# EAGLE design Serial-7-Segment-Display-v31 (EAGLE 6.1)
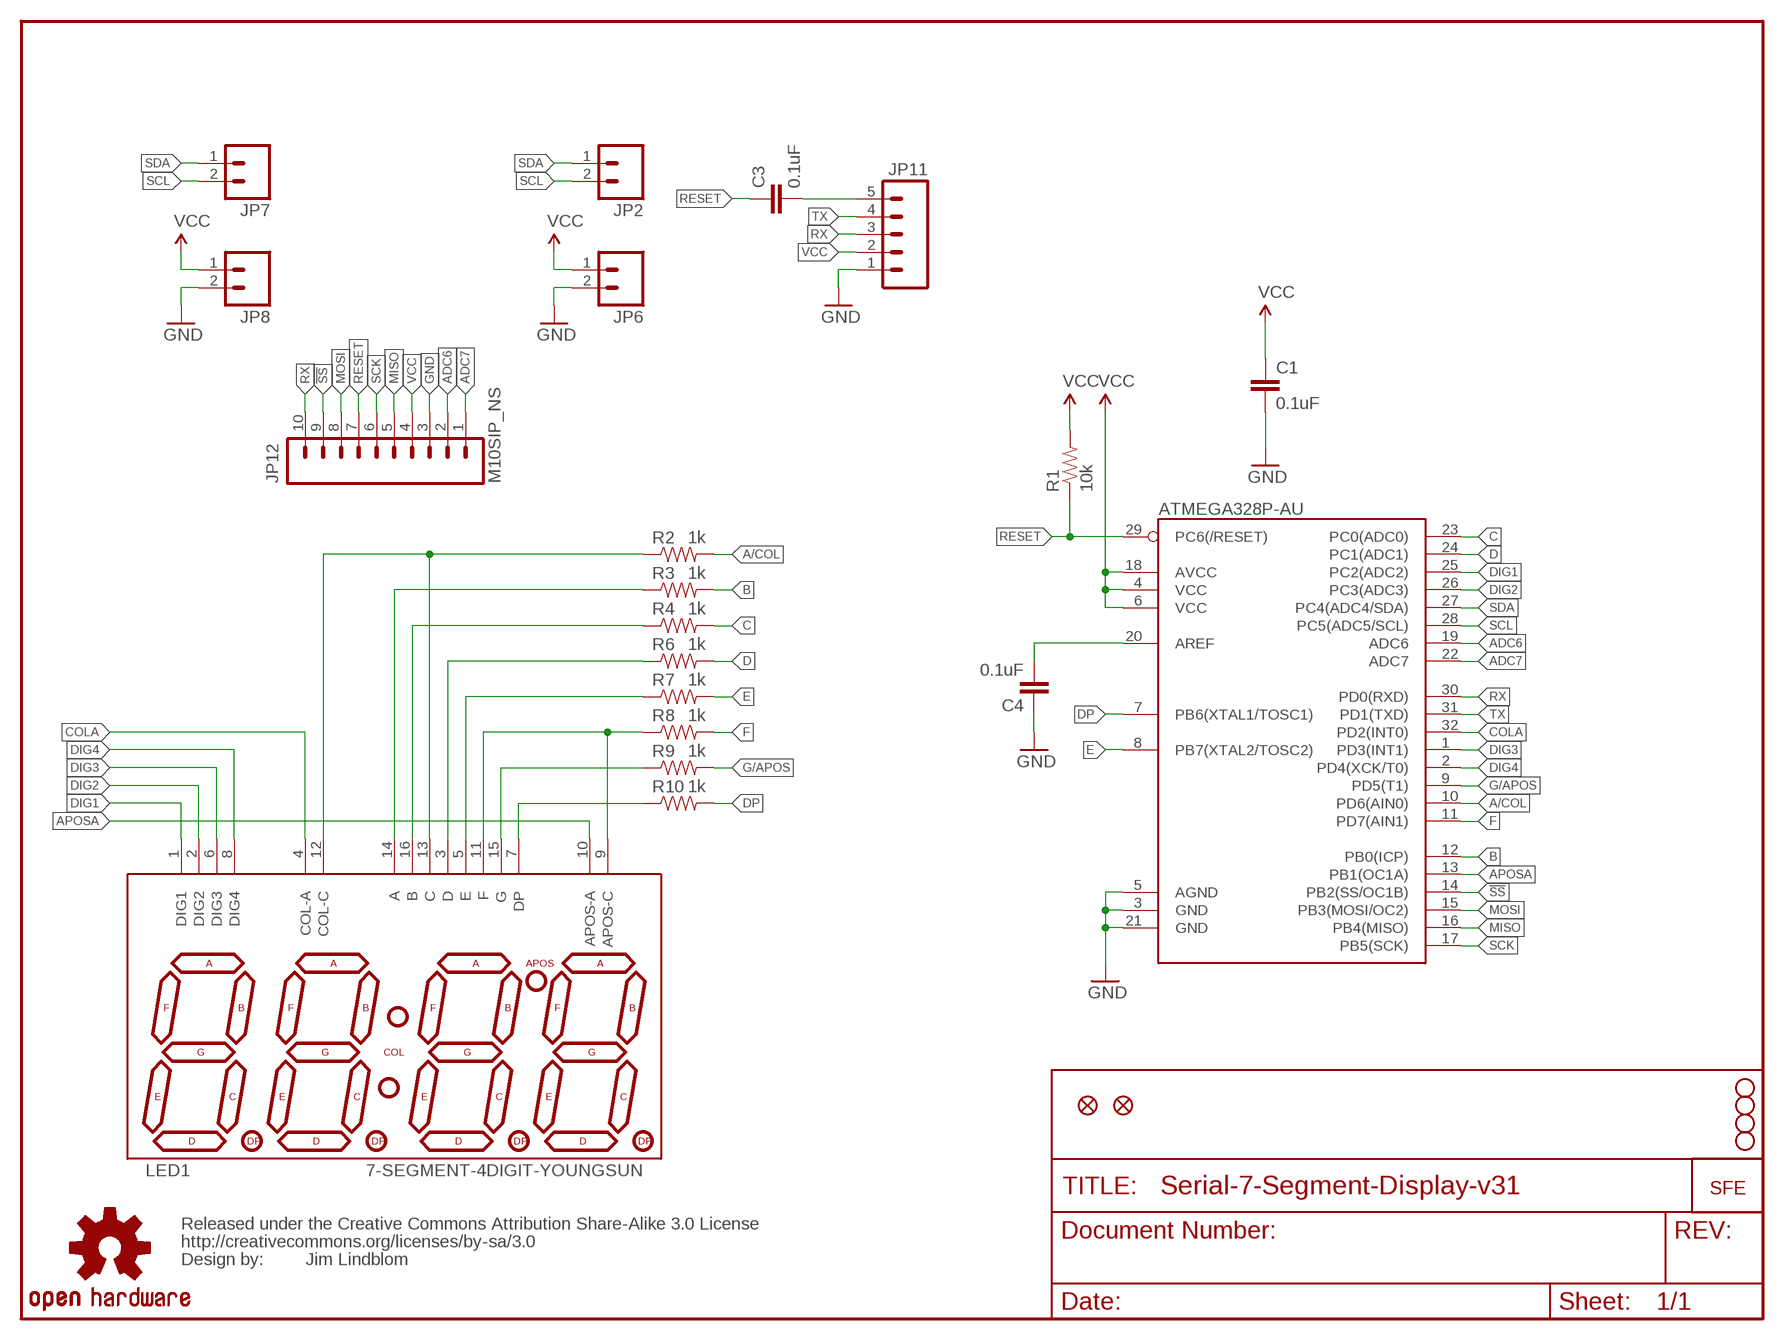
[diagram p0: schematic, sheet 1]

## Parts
ATMEGA328P-AU  ATMEGA328P-AU  ATMEGA168  [TQFP32-08]
C1  0.1uF  CAP0402-CAP  [0402-CAP]
C3  0.1uF  CAP0402-CAP  [0402-CAP]
C4  0.1uF  CAP0402-CAP  [0402-CAP]
JP1  STAND-OFF  [STAND-OFF]
JP2  M021X02_NO_SILK  [1X02_NO_SILK]
JP3  STAND-OFF  [STAND-OFF]
JP4  STAND-OFF  [STAND-OFF]
JP5  STAND-OFF  [STAND-OFF]
JP6  M021X02_NO_SILK  [1X02_NO_SILK]
JP7  M021X02_NO_SILK  [1X02_NO_SILK]
JP8  M021X02_NO_SILK  [1X02_NO_SILK]
JP9  FIDUCIALUFIDUCIAL  [MICRO-FIDUCIAL]
JP10  FIDUCIALUFIDUCIAL  [MICRO-FIDUCIAL]
JP11  M05PTH-NS  [1X05_NO_SILK]
JP12  M10SIP_NS  [1X10_NO_SILK]
LED1  7-SEGMENT-4DIGIT-YOUNGSUN  [7-SEGMENT-4DIGIT-YOUNGSUN]
R1  10k  RESISTOR0402-RES  [0402-RES]
R2  1k  RESISTOR0402-RES  [0402-RES]
R3  1k  RESISTOR0402-RES  [0402-RES]
R4  1k  RESISTOR0402-RES  [0402-RES]
R6  1k  RESISTOR0402-RES  [0402-RES]
R7  1k  RESISTOR0402-RES  [0402-RES]
R8  1k  RESISTOR0402-RES  [0402-RES]
R9  1k  RESISTOR0402-RES  [0402-RES]
R10  1k  RESISTOR0402-RES  [0402-RES]
U$1  CREATIVE_COMMONS  [CREATIVE_COMMONS]
U$2  LOGO-SFESK  [SFE-LOGO-FLAME]
U$4  OSHW-LOGOS  [OSHW-LOGO-S]

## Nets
!SS: ATMEGA328P-AU.14(PB2(SS/OC1B)) JP12.9
A/COL: ATMEGA328P-AU.10(PD6(AIN0)) R2.2
ADC6: ATMEGA328P-AU.19(ADC6) JP12.2
ADC7: ATMEGA328P-AU.22(ADC7) JP12.1
APOSA: ATMEGA328P-AU.13(PB1(OC1A)) LED1.10(APOS-A)
B: ATMEGA328P-AU.12(PB0(ICP)) R3.2
C: ATMEGA328P-AU.23(PC0(ADC0)) R4.2
COLA: ATMEGA328P-AU.32(PD2(INT0)) LED1.4(COL-A)
D: ATMEGA328P-AU.24(PC1(ADC1)) R6.2
DIG1: ATMEGA328P-AU.25(PC2(ADC2)) LED1.1(DIG1)
DIG2: ATMEGA328P-AU.26(PC3(ADC3)) LED1.2(DIG2)
DIG3: ATMEGA328P-AU.1(PD3(INT1)) LED1.6(DIG3)
DIG4: ATMEGA328P-AU.2(PD4(XCK/T0)) LED1.8(DIG4)
DP: ATMEGA328P-AU.7(PB6(XTAL1/TOSC1)) R10.2
E: ATMEGA328P-AU.8(PB7(XTAL2/TOSC2)) R7.2
F: ATMEGA328P-AU.11(PD7(AIN1)) R8.2
G/APOS: ATMEGA328P-AU.9(PD5(T1)) R9.2
GND: ATMEGA328P-AU.3(GND) ATMEGA328P-AU.5(AGND) ATMEGA328P-AU.21(GND) C1.2 C4.1 JP6.2 JP8.2 JP11.1 JP12.3
MISO: ATMEGA328P-AU.16(PB4(MISO)) JP12.5
MOSI: ATMEGA328P-AU.15(PB3(MOSI/OC2)) JP12.8
N$1: ATMEGA328P-AU.20(AREF) C4.2
N$2: LED1.7(DP) R10.1
N$3: LED1.15(G) R9.1
N$4: LED1.9(APOS-C) LED1.11(F) R8.1
N$5: LED1.5(E) R7.1
N$6: LED1.3(D) R6.1
N$8: LED1.16(B) R4.1
N$9: LED1.14(A) R3.1
N$10: LED1.12(COL-C) LED1.13(C) R2.1
N$13: C3.2 JP11.5
RESET: ATMEGA328P-AU.29(PC6(/RESET)) C3.1 JP12.7 R1.1
RX: ATMEGA328P-AU.30(PD0(RXD)) JP11.3 JP12.10
SCK: ATMEGA328P-AU.17(PB5(SCK)) JP12.6
SCL: ATMEGA328P-AU.28(PC5(ADC5/SCL)) JP2.2 JP7.2
SDA: ATMEGA328P-AU.27(PC4(ADC4/SDA)) JP2.1 JP7.1
TX: ATMEGA328P-AU.31(PD1(TXD)) JP11.4
VCC: ATMEGA328P-AU.4(VCC) ATMEGA328P-AU.6(VCC) ATMEGA328P-AU.18(AVCC) C1.1 JP6.1 JP8.1 JP11.2 JP12.4 R1.2

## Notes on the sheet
- Jim Lindblom

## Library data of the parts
ATMEGA328P-AU = SparkFun:ATMEGA168
C1 = SparkFun:CAP: Capacitor
C3 C4 = SparkFun-Passives:CAP: Capacitor
JP1 JP3-JP5 = SparkFun-Electromechanical:STAND-OFF: #4 Stand Off
JP2 JP6-JP8 = SparkFun-Connectors:M02: Header 2
JP9 JP10 = SparkFun:FIDUCIAL: Fiducial Alignment Points
JP11 = SparkFun-Connectors:M05: Header 5 Standard 5-pin 0.1" header. Use with straight break away headers (SKU : PRT-00116), right angle break away headers (PRT-00553), swiss pins (PRT-00743), machine pins (PRT-00117), and female headers (PRT-00115). Molex polarized connector foot print use with SKU : PRT-08230 with associated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
JP12 = SparkFun-Connectors:M10: Header 10 Standard 10-pin 0.1" header. Use with straight break away headers (SKU : PRT-00116), right angle break away headers (PRT-00553), swiss pins (PRT-00743), machine pins (PRT-00117), and female headers (PRT-00115).
LED1 = SparkFun:7-SEGMENT-4DIGIT-YOUNGSUN: This is a part for the 4-Digit 7-segment LEDs from Young Sun. Different from the Digikey LEDs, all 16 pins are used. The LONGPADS Variant is used for a test jig, but you may like it because there is more pad to solder to. If you are concerned about routing space, the standard works just fine though.
R1-R4 R6-R10 = SparkFun:RESISTOR: Resistor
U$1 = SparkFun:CREATIVE_COMMONS
U$2 = SparkFun:LOGO-SFE: Spark Fun Electronics PCB Logo
U$4 = SparkFun-Aesthetics:OSHW-LOGO: Open Source Hardware Logo This logo indicates the piece of hardware it is found on incorporates a OSHW license and/or adheres to the definition of open source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

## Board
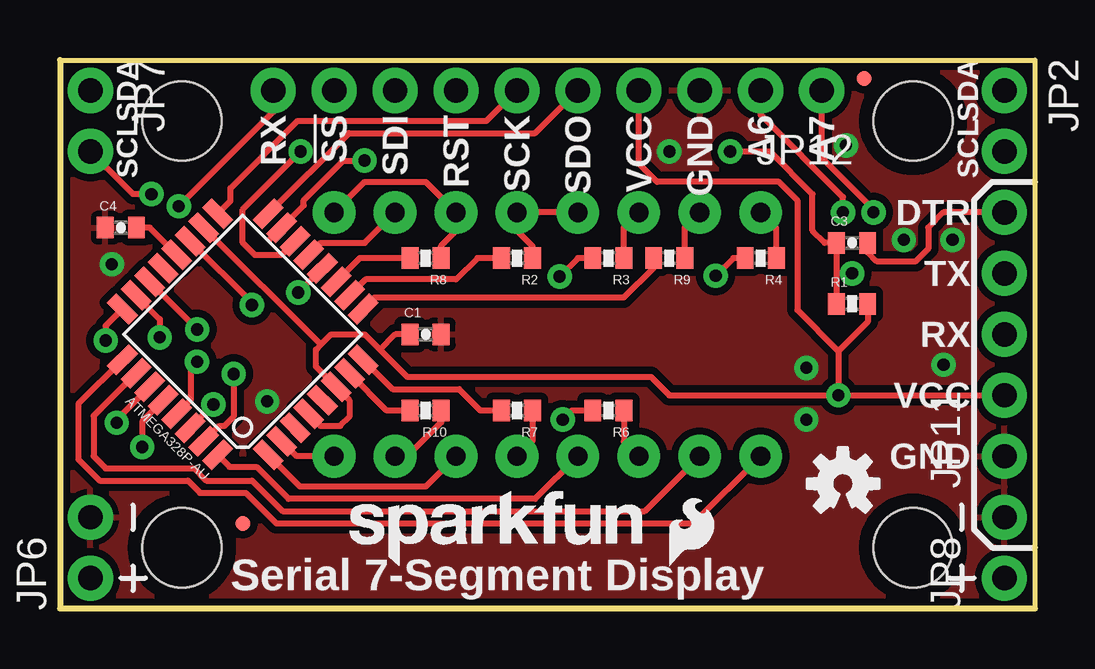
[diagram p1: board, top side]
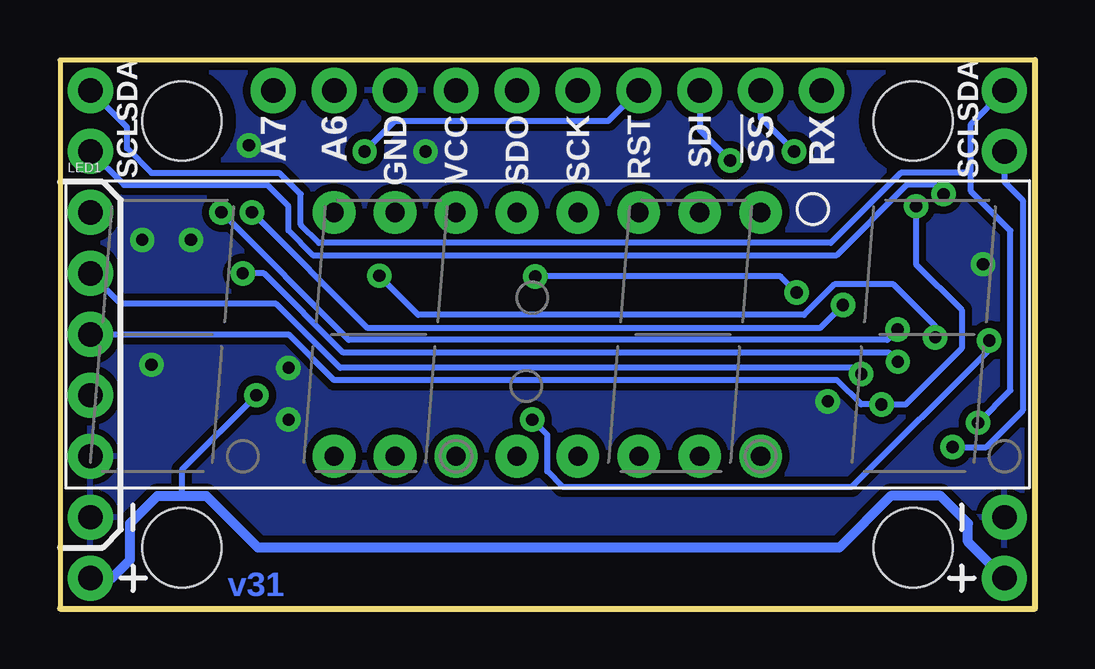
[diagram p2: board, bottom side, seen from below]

Size 40.64 x 22.86 mm. Coordinates in mm from the lower left corner, seen from the top.
Outline: 0,22.86 40.64,22.86 40.64,0 0,0 0,22.86
Copper layers (1*16): Top 0.035mm / dielectric 1.5mm / Bottom 0.035mm
Design rules: minimum track width 8mil, minimum drill 20mil, track to track 8mil, track to pad 8mil, pad to pad 8mil, via to via 8mil, smd to smd 8mil, copper to edge 8mil, drill to drill 8mil, minimum pad ring 12mil, minimum via ring 10mil, stop-mask expansion 4mil, vias tented up to drill 20mil, thermal gap 10mil

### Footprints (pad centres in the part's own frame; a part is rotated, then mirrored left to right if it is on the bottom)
TQFP32-08 = smd 1.27 x 0.559: 1 -4.293,2.8; 2 -4.293,2; 3 -4.293,1.2; 4 -4.293,0.4; 5 -4.293,-0.4; 6 -4.293,-1.2; 7 -4.293,-2; 8 -4.293,-2.8; 17 4.293,-2.8; 18 4.293,-2; 19 4.293,-1.2; 20 4.293,-0.4; 21 4.293,0.4; 22 4.293,1.2; 23 4.293,2; 24 4.293,2.8 | smd 0.559 x 1.27: 9 -2.8,-4.293; 10 -2,-4.293; 11 -1.2,-4.293; 12 -0.4,-4.293; 13 0.4,-4.293; 14 1.2,-4.293; 15 2,-4.293; 16 2.8,-4.293; 25 2.8,4.293; 26 2,4.293; 27 1.2,4.293; 28 0.4,4.293; 29 -0.4,4.293; 30 -1.2,4.293; 31 -2,4.293; 32 -2.8,4.293
0402-CAP = smd 0.7 x 0.9: 1 -0.65,0; 2 0.65,0
STAND-OFF = hole 3.302: 0,0
1X02_NO_SILK = drill 1.016 pad 1.88: 1 0,0; 2 2.54,0
MICRO-FIDUCIAL = smd 0.635 x 0.635: 1 0,0
1X05_NO_SILK = drill 1.016 pad 1.88: 1 0,0; 2 2.54,0; 3 5.08,0; 4 7.62,0; 5 10.16,0
1X10_NO_SILK = drill 1.016 pad 1.88: 1 0,0; 2 2.54,0; 3 5.08,0; 4 7.62,0; 5 10.16,0; 6 12.7,0; 7 15.24,0; 8 17.78,0; 9 20.32,0; 10 22.86,0
7-SEGMENT-4DIGIT-YOUNGSUN = drill 0.8 pad 1.778: 1 -8.89,-5.08; 2 -6.35,-5.08; 3 -3.81,-5.08; 4 -1.27,-5.08; 5 1.27,-5.08; 6 3.81,-5.08; 7 6.35,-5.08; 8 8.89,-5.08; 9 8.89,5.08; 10 6.35,5.08; 11 3.81,5.08; 12 1.27,5.08; 13 -1.27,5.08; 14 -3.81,5.08; 15 -6.35,5.08; 16 -8.89,5.08
0402-RES = smd 0.7 x 0.9: 1 -0.65,0; 2 0.65,0

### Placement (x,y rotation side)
ATMEGA328P-AU  7.62,11.43 135 top
C1  15.24,11.43 0 top
C3  33.02,15.24 0 top
C4  2.54,15.88 0 top
JP1  5.08,2.54 0 top
JP2  39.37,21.59 270 top
JP3  5.08,20.32 0 top
JP4  35.56,2.54 0 top
JP5  35.56,20.32 0 top
JP6  1.27,1.27 90 top
JP7  1.27,21.59 270 top
JP8  39.37,1.27 90 top
JP9  33.53,22.1 0 top
JP10  7.62,3.56 0 top
JP11  39.37,6.35 90 top
JP12  31.75,21.59 180 top
LED1  20.32,11.43 0 bottom
R1  33.02,12.7 0 top
R2  19.05,14.61 180 top
R3  22.86,14.61 180 top
R4  29.21,14.61 180 top
R6  22.86,8.26 180 top
R7  19.05,8.26 180 top
R8  15.24,14.61 180 top
R9  25.4,14.61 180 top
R10  15.24,8.26 180 top
U$1  not placed on the board
U$2  25.4,1.78 0 top
U$3  LOGO-SFENW2  [SFE-NEW-WEB]  12.06,1.78 0 top
U$4  32.64,5.21 0 top

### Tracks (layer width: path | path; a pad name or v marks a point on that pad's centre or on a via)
!SS  (via drill 0.51)
  Top 0.254: ATMEGA328P-AU.14 9.22,14.73 8.13,14.73 7.62,15.24 7.62,16.64 v10.03,19.05
  Bottom 0.254: v10.03,19.05 11.43,20.45 JP12.9
A/COL
  Top 0.254: R2.2 17.4,14.61 16.51,13.72 12.73,13.72 ATMEGA328P-AU.10
ADC6  (via drill 0.51)
  Top 0.254: ATMEGA328P-AU.19 8,12.75 v8,12.65 | v32.64,16.51 32.64,17.14 29.21,20.57 JP12.2
  Bottom 0.254: v32.64,16.51 27.81,11.68 8.97,11.68 v8,12.65
ADC7  (via drill 0.51)
  Top 0.254: JP12.1 31.75,18.8 33.91,16.64 v33.91,16.51 | ATMEGA328P-AU.22 v5.72,11.63
  Bottom 0.254: v33.91,16.51 28.6,11.2 6.15,11.2 v5.72,11.63
APOSA
  Top 0.254: LED1.10 12.7,15.24 10.86,15.24 ATMEGA328P-AU.13
B  (via drill 0.51)
  Top 0.254: R3.2 21.59,14.61 v20.83,13.84 | ATMEGA328P-AU.12 v9.93,13.18
  Bottom 0.254: v9.93,13.18 10.6,13.84 v20.83,13.84
C  (via drill 0.51)
  Top 0.254: ATMEGA328P-AU.23 4.16,12.06 v4.16,11.3 | R4.2 28.07,14.61 v27.33,13.87
  Bottom 0.254: v4.16,11.3 4.16,11.78 5.89,13.51 8.36,13.51 9.63,12.24 25.7,12.24 v27.33,13.87
COLA
  Top 0.254: LED1.4 19.81,4.57 9.53,4.57 8.19,5.91 7.07,5.91 ATMEGA328P-AU.32
D  (via drill 0.51)
  Top 0.254: ATMEGA328P-AU.24 1.91,11.79 v1.91,11.18 | R6.2 21.34,8.26 v20.95,7.87
  Bottom 0.254: v20.95,7.87 20.32,7.24 20.32,5.71 19.68,5.08 7.62,5.08 1.91,10.79 v1.91,11.18
DIG1
  Top 0.254: ATMEGA328P-AU.25 0.76,8.53 0.76,6.22 1.65,5.33 5.33,5.33 5.84,4.83 7.75,4.83 9.02,3.56 26.42,3.56 LED1.1
DIG2
  Top 0.254: ATMEGA328P-AU.26 1.4,8.04 1.4,6.35 1.91,5.84 5.59,5.84 6.1,5.33 8,5.33 9.27,4.06 24.38,4.06 LED1.2
DIG3
  Top 0.254: LED1.6 15.24,5.08 10.01,5.08 ATMEGA328P-AU.1
DIG4
  Top 0.254: LED1.8 9.87,6.35 ATMEGA328P-AU.2
DP
  Top 0.254: ATMEGA328P-AU.7 13.62,8.26 R10.2
E
  Top 0.254: ATMEGA328P-AU.8 13.87,9.14 16.64,9.14 17.53,8.26 R7.2
F
  Top 0.254: R8.2 12.49,14.61 ATMEGA328P-AU.11
G/APOS
  Top 0.254: R9.2 24.75,14.21 23.5,12.95 13.1,12.95 ATMEGA328P-AU.9
GND  (via drill 0.51)
  other vias: 31.11,7.87 2.16,14.35 37.21,15.37 36.83,10.16 31.11,10.03 8.64,8.64 25.4,19.05 32.77,19.3 35.18,15.37
  pour Top (isolate 0.305): 0,0 0,22.86 40.64,22.86 40.64,0
  pour Bottom (isolate 0.305): 0,0 0,22.86 40.64,22.86 40.64,0
MISO
  Top 0.254: ATMEGA328P-AU.16 12.04,19.81 19.81,19.81 JP12.5
MOSI  (via drill 0.51)
  Top 0.254: 8.73,15.37 ATMEGA328P-AU.15 10.16,16.8 10.16,17.02 11.81,18.67 v12.7,18.67
  Bottom 0.254: JP12.8 13.97,19.94 v12.7,18.67
N$1
  Top 0.254: ATMEGA328P-AU.20 3.74,15.88 C4.2
N$2
  Top 0.254: LED1.7 14.48,6.35 15.89,7.76 R10.1
N$3
  Top 0.254: R9.1 26.05,15.89 LED1.15
N$4
  Top 0.254: R8.1 15.89,15.13 16.51,15.75 LED1.11 15.24,17.78 12.7,17.78 LED1.9
N$5
  Top 0.254: R7.1 19.7,7 LED1.5
N$6
  Top 0.254: R6.1 23.51,6.97 LED1.3
N$8
  Top 0.254: R4.1 29.86,15.86 LED1.16
N$9
  Top 0.254: R3.1 23.51,15.89 LED1.14
N$10
  Top 0.254: R2.1 19.7,15.1 19.05,15.75 LED1.12 LED1.13
N$13
  Top 0.254: JP11.5 36.83,16.51 36.2,15.88 36.2,14.99 35.69,14.48 34.04,14.48 33.67,14.84 C3.2
RESET  (via drill 0.51)
  Top 0.254: ATMEGA328P-AU.29 5.46,8.71 5.46,10.03 v5.71,10.29 | 32.37,13.97 C3.1 31.88,15.24 31.37,15.75 31.37,17.27 29.59,19.05 v27.94,19.05 | 32.37,13.97 R1.1 | v33.02,13.97 32.37,13.97
  Bottom 0.254: v27.94,19.05 26.67,20.32 17.78,20.32 JP12.7 | v33.02,13.97 32.13,13.97 28.83,10.67 6.1,10.67 v5.71,10.29
RX  (via drill 0.51)
  Top 0.254: ATMEGA328P-AU.30 v6.4,8.51 | JP12.10 8.89,20.7 v4.95,16.76
  Bottom 0.254: JP11.3 31.11,11.43 29.21,9.53 8.26,9.53 7.24,8.51 v6.4,8.51 | v4.95,16.76 4.95,14.35 3.05,12.45 3.05,10.84 5.38,8.51 v6.4,8.51 | v6.4,8.51 6.73,8.51
SCK
  Top 0.254: ATMEGA328P-AU.17 7.11,16.99 7.11,17.53 9.91,20.32 17.78,20.32 JP12.6
SCL  (via drill 0.51)
  Top 0.254: ATMEGA328P-AU.28 3.43,7.8 v3.43,6.73 | v3.81,17.27 3.05,17.27 JP7.2
  Bottom 0.254: JP7.2 1.27,17.78 0.51,17.02 0.51,8.26 2.03,6.73 v3.43,6.73 | JP2.2 37.97,17.65 32,17.65 31.11,16.76 31.11,15.75 30.1,14.73 8.26,14.73 5.33,17.65 4.19,17.65 v3.81,17.27
SDA  (via drill 0.51)
  Top 0.254: ATMEGA328P-AU.27 2.37,7.87 v2.37,7.75
  Bottom 0.254: v2.37,7.75 1.02,9.1 1.02,15.75 2.67,17.4 2.67,18.16 | 2.67,18.16 2.67,20.19 JP7.1 | JP2.1 37.85,20.07 37.85,19.18 36.83,18.16 31.5,18.16 30.61,17.27 30.61,16 29.84,15.24 8.51,15.24 5.59,18.16 2.67,18.16
TX  (via drill 0.51)
  Top 0.254: ATMEGA328P-AU.31 6.64,7.62 6.86,7.62 7.24,8 v7.24,9.78
  Bottom 0.254: v7.24,9.78 7.49,10.03 28.96,10.03 31.62,12.7 38.1,12.7 JP11.4
VCC  (via drill 0.51)
  Top 0.254: ATMEGA328P-AU.18 10.86,11.02 10.86,10.99 | 32.45,10.73 30.73,12.45 30.73,17.02 29.97,17.78 24.89,17.78 24.13,18.54 JP12.4 | R1.2 33.67,11.95 32.45,10.73 | 13.34,10.79 12.7,11.43 11.3,11.43 10.86,10.99 | 13.34,10.79 14.48,9.65 24.64,9.65 25.4,8.89 v32.45,8.89 | C1.1 13.97,11.43 13.34,10.79 | ATMEGA328P-AU.4 10.86,7.62 11.68,7.62 12.06,8 12.06,8.68 ATMEGA328P-AU.6 10.67,10.08 10.67,10.79 10.86,10.99 | 32.45,10.73 v32.45,8.89 | v32.45,8.89 JP11.2
  Bottom 0.254: v32.45,8.89 35.56,5.78 35.56,4.7
  Bottom 0.406: JP6.1 2.79,2.79 2.79,3.56 3.94,4.7 5.99,4.7 8.15,2.54 32.38,2.54 34.54,4.7 35.56,4.7 36.58,4.7 37.72,3.56 37.72,2.03 38.48,1.27 JP8.1

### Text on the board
Bottom: v31
tPlace: SDA | SDA | RX | !SS | SDI | RST | SCK | SDO | VCC | GND | A6 | A7 | SCL | SCL | DTR | TX | RX | VCC | GND | Serial 7-Segment Display
bPlace: SDA | SDA | RX | !SS | SDI | RST | SCK | SDO | VCC | GND | A6 | A7 | SCL | SCL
